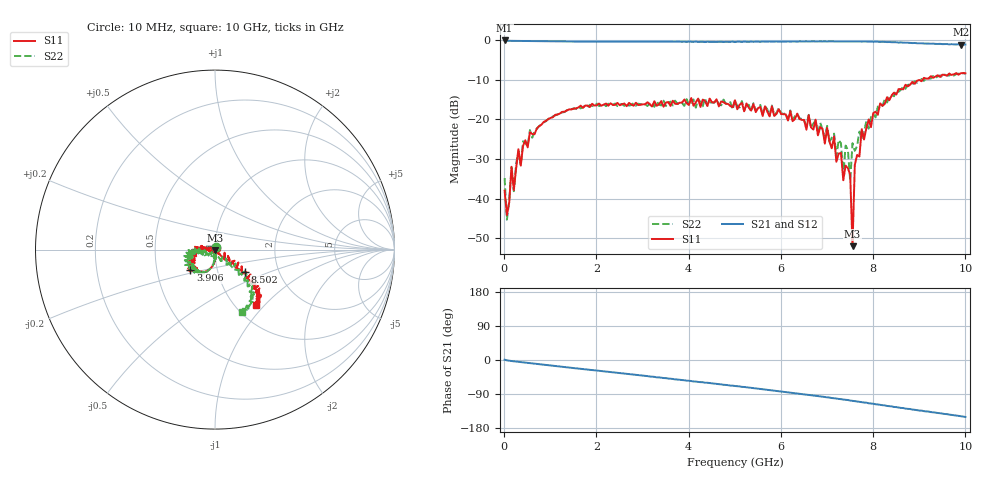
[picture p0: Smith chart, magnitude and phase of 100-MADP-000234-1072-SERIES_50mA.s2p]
!Agilent Technologies,E8364C,MY48140145,A.09.42.15
!Agilent E8364C: A.09.42.15
!Date: Wednesday, December 02, 2020 08:32:39
!Correction: S11(Full 2 Port(1,2))
!S21(Full 2 Port(1,2))
!S12(Full 2 Port(1,2))
!S22(Full 2 Port(1,2))
!S2P File: Measurements: S11, S21, S12, S22:
# Hz S  dB  R 50
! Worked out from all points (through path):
!   201 points, 10 MHz to 10 GHz, reference 50 ohm
!   highest |S21| = -0.02 dB at 10 MHz (marker M1); lowest = -1.1 dB at 9.9 GHz (marker M2)
!   group delay of S21, straight-line fit = 41 ps
!   lowest |S11| = -52.0 dB at 7.552 GHz (marker M3), VSWR 1.01, Z = 49.8 - j0.17 ohm
!   |S11| at or under -10 dB: start of sweep to 9.071 GHz
!   |S22| runs from -45.4 to -8.2 dB; largest |S21 - S12| = 0.019
!   S11 on the Smith chart (normalised r, x): 10 MHz: 1.01, +0.02; 3.906 GHz: 0.74, -0.17; 8.502 GHz: 1.35, -0.34; 10 GHz: 1.24, -0.89
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1e7  -37.99 56.3  -0.02 0.8  -0.03 -0.3  -34.84 67.0
5.995e7  -44.16 -64.0  -0.10 -1.0  -0.10 -1.1  -45.36 -78.5
1.5985e8  -31.96 -77.0  -0.12 -2.7  -0.11 -2.7  -32.22 -75.0
2.098e8  -37.85 -70.3  -0.13 -3.5  -0.12 -3.5  -38.14 -78.5
3.097e8  -27.51 -85.7  -0.15 -4.9  -0.15 -4.9  -27.93 -81.8
5.5945e8  -23.24 -93.4  -0.20 -8.5  -0.19 -8.6  -22.69 -90.7
1.7083e9  -17.07 -118.9  -0.32 -24.0  -0.30 -23.9  -16.87 -117.6
3.35665e9  -16.18 -137.7  -0.30 -46.0  -0.31 -46.1  -16.29 -127.3
3.9061e9  -14.97 -140.4  -0.34 -53.4  -0.36 -54.0  -16.59 -135.7
5.005e9  -15.13 -151.0  -0.43 -68.6  -0.38 -68.5  -15.14 -168.3
6.7033e9  -22.55 172.0  -0.26 -93.9  -0.23 -93.5  -21.04 175.5
7.15285e9  -24.30 167.3  -0.27 -100.9  -0.29 -101.3  -23.59 -151.0
7.35265e9  -35.38 -100.9  -0.26 -104.4  -0.23 -104.0  -34.17 -141.8
7.4026e9  -31.67 148.6  -0.26 -105.1  -0.25 -105.2  -26.60 -137.3
7.5025e9  -34.01 -46.3  -0.26 -107.0  -0.23 -106.5  -35.55 -113.8
7.55245e9  -52.05 -137.0  -0.27 -107.7  -0.27 -108.0  -26.01 -95.7
7.6024e9  -31.51 -47.6  -0.26 -108.5  -0.25 -108.5  -27.92 -73.4
7.75225e9  -22.44 -44.6  -0.30 -111.3  -0.25 -110.9  -24.95 -38.6
8.35165e9  -15.15 -31.9  -0.42 -121.9  -0.44 -121.9  -14.27 -46.7
8.5015e9  -13.71 -36.3  -0.47 -124.3  -0.51 -124.7  -12.69 -44.7
9.9001e9  -8.31 -54.2  -1.09 -148.3  -1.01 -148.3  -8.78 -64.7
1e10  -8.33 -53.4  -1.06 -150.3  -1.06 -150.3  -8.44 -66.9
